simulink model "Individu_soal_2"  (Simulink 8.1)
settings: Solver=ode45  StartTime=0.0  StopTime=3.0  RelTol=1e-3

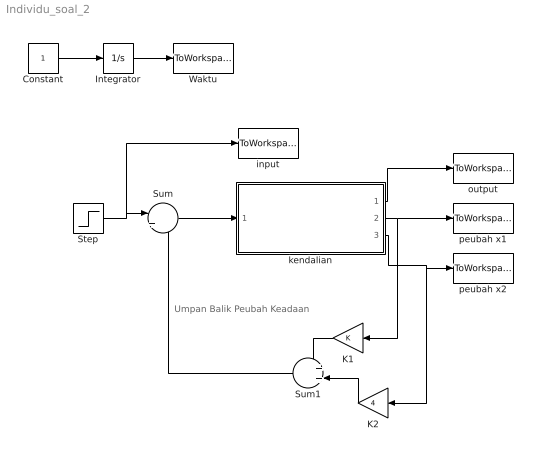
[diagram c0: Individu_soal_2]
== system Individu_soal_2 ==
  note: Umpan Balik Peubah Keadaan
  Constant : Constant
  Integrator : Integrator
  K1 : Gain
  K2 : Gain  Gain=4
  Step : Step  SampleTime=0
  Sum : Sum  Inputs=|+-
  Sum1 : Sum
  Waktu : ToWorkspace  VariableName=time  SampleTime=-1
  input : ToWorkspace  VariableName=u  SampleTime=-1
  kendalian : Subsystem
  output : ToWorkspace  VariableName=y  SampleTime=-1
  peubah x1 : ToWorkspace  VariableName=x1  SampleTime=-1
  peubah x2 : ToWorkspace  VariableName=x2  SampleTime=-1
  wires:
  Constant/1 -> Integrator/1
  Integrator/1 -> Waktu/1
  kendalian/1(y) -> output/1
  Step/1 -> Sum/1, input/1
  kendalian/2(x1) -> K1/1, peubah x1/1
  kendalian/3(x2) -> K2/1, peubah x2/1
  K1/1 -> Sum1/1
  K2/1 -> Sum1/2
  Sum1/1 -> Sum/2
  Sum/1 -> kendalian/1(u)

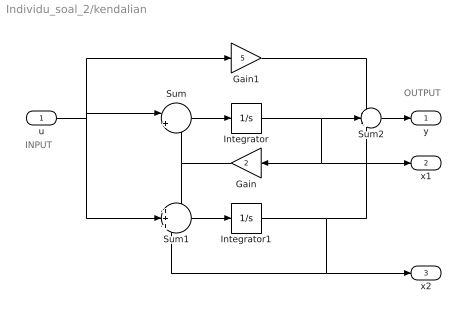
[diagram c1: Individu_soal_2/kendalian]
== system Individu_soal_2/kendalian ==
  note: INPUT
  note: OUTPUT
  u : Inport
  Gain : Gain  Gain=2
  Gain1 : Gain  Gain=5
  Integrator : Integrator
  Integrator1 : Integrator
  Sum : Sum  Inputs=|++
  Sum1 : Sum  Inputs=+++
  Sum2 : Sum  Inputs=+++
  y : Outport
  x1 : Outport  Port=2
  x2 : Outport  Port=3
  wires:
  Integrator/1 -> x1/1, Gain/1, Sum2/2
  Integrator1/1 -> x2/1, Sum1/3, Sum2/3
  u/1 -> Sum1/2, Sum/1, Gain1/1
  Sum/1 -> Integrator/1
  Gain/1 -> Sum1/1, Sum/2
  Sum1/1 -> Integrator1/1
  Sum2/1 -> y/1
  Gain1/1 -> Sum2/1
